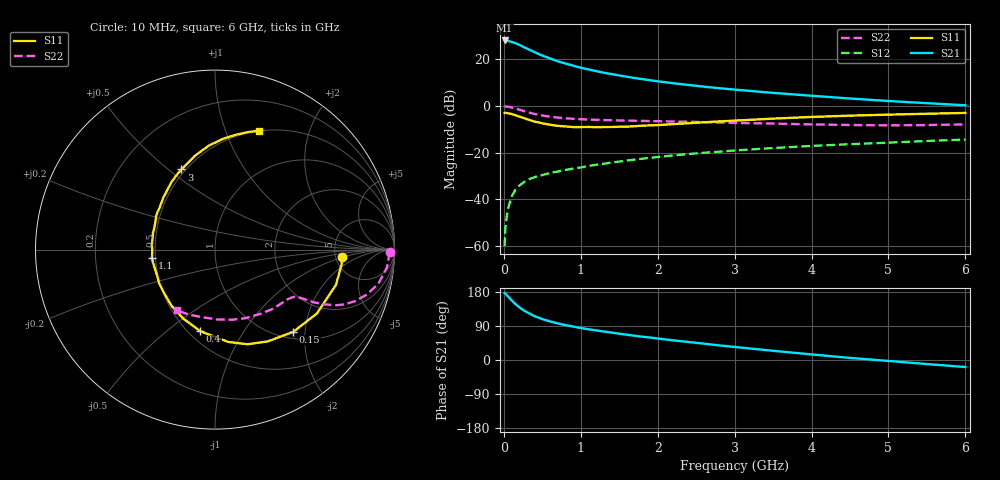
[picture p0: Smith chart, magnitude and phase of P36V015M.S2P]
! SIEMENS Small Signal Semiconductors
! BFP181
! Si NPN RF Bipolar Junction Transistor in SOT143
! VCE = 6 V  IC = 15 mA
! Common Emitter S-Parameters:  March  1996
# GHz  S  MA  R  50
!  f  S11  S21  S12  S22
! GHz  MAG  ANG  MAG  ANG  MAG  ANG  MAG  ANG
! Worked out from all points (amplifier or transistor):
!   36 points, 10 MHz to 6 GHz, reference 50 ohm
!   highest |S21| = 28.0 dB at 10 MHz (marker M1)
!   |S21| within 3 dB of that: start of sweep to 269.5 MHz
!   unconditionally stable (mu >= 1): 980.2 MHz to end of sweep
!   at 250 MHz: K = 0.40, MSG = 29.1 dB, |S12| = -32.9 dB
!   at 1.4 GHz: K = 1.10, MAG = 17.0 dB, |S12| = -24.2 dB
!   at 6 GHz: K = 1.00, MAG = 7.0 dB, |S12| = -14.4 dB
!   S11 on the Smith chart (normalised r, x): 10 MHz: 5.66, -0.89; 150 MHz: 1.14, -1.74; 400 MHz: 0.57, -0.66; 1.1 GHz: 0.48, -0.05; 3 GHz: 0.48, +0.56; 6 GHz: 0.50, +1.31
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0.01  0.7059 -3.2  25.08 176.9  0.001 70.0  0.973 -0.8
0.02  0.7101 -6.6  24.9 175.3  0.0025 88.6  0.9704 -2.2
0.05  0.7022 -16.2  24.72 168.5  0.006 84.3  0.9624 -6.1
0.1  0.6702 -32.0  23.37 157.8  0.0114 74.9  0.9299 -11.8
0.15  0.6325 -46.4  21.91 147.8  0.0161 69.5  0.8831 -16.4
0.2  0.5906 -59.9  20.22 139.3  0.0197 64.9  0.8331 -20.1
0.25  0.5577 -71.0  18.37 132.0  0.0227 61.1  0.7842 -22.9
0.3  0.52 -81.8  16.83 126.1  0.0259 58.3  0.742 -24.7
0.4  0.4621 -100.2  14.08 115.6  0.03 55.2  0.672 -26.9
0.5  0.4232 -114.7  11.9 107.9  0.0332 52.6  0.6218 -28.1
0.6  0.3957 -127.7  10.36 101.9  0.0368 52.6  0.5874 -28.7
0.7  0.3739 -138.8  8.999 96.7  0.0394 52.4  0.5626 -29.1
0.9  0.3524 -157.2  7.252 88.2  0.0457 52.3  0.5297 -29.9
1.1  0.3549 -172.4  6.028 81.0  0.052 52.6  0.5107 -31.1
1.3  0.3531 175.3  5.117 75.1  0.0579 52.8  0.4979 -32.9
1.6  0.3602 159.3  4.2 66.7  0.0679 52.0  0.4854 -36.0
2.2  0.4079 135.1  3.051 51.9  0.0871 49.2  0.464 -43.9
3  0.484 112.7  2.231 34.4  0.1111 43.5  0.4333 -56.7
3.5  0.5343 102.1  1.896 24.3  0.1254 39.9  0.418 -66.2
4.5  0.6185 85.9  1.438 5.5  0.1518 31.5  0.3899 -87.8
5.5  0.6792 74.4  1.142 -10.7  0.1778 24.2  0.3891 -110.6
6  0.7068 69.7  1.031 -18.5  0.1903 20.2  0.401 -122.3
